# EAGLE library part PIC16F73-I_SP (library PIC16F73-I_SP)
8-bit CMOS FLASH Microcontrollers Source: Datasheet
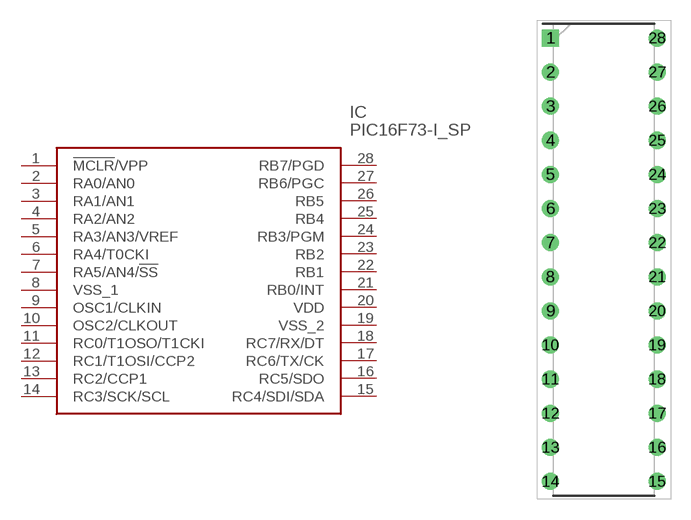
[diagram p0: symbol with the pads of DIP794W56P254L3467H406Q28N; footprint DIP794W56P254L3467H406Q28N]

Designator prefix IC

## PIC16F73-I_SP (Description: 8-bit CMOS FLASH Microcontrollers; Height: 4.06mm; Manufacturer_Name: Microchip; Manufacturer_Part_Number: PIC16F73-I/SP; Mouser_Part_Number: 579-PIC16F73ISP; Mouser_Price-Stock: https://www.mouser.co.uk/ProductDetail/Microchip-Technology-Atmel/PIC16F73-I-SP?qs=BJWliqx2vnXd6B3M0zIKjg%3D%3D)  [DIP794W56P254L3467H406Q28N]
1  !MCLR!/VPP
2  RA0/AN0
3  RA1/AN1
4  RA2/AN2
5  RA3/AN3/VREF
6  RA4/T0CKI
7  RA5/AN4/!SS
8  VSS_1
9  OSC1/CLKIN
10  OSC2/CLKOUT
11  RC0/T1OSO/T1CKI
12  RC1/T1OSI/CCP2
13  RC2/CCP1
14  RC3/SCK/SCL
15  RC4/SDI/SDA
16  RC5/SDO
17  RC6/TX/CK
18  RC7/RX/DT
19  VSS_2
20  VDD
21  RB0/INT
22  RB1
23  RB2
24  RB3/PGM
25  RB4
26  RB5
27  RB6/PGC
28  RB7/PGD

## Footprint DIP794W56P254L3467H406Q28N (pad centres in mm)
28 PDIP
drill 0.76 pad 1.16 square: 1 -3.97,16.51
drill 0.76 pad 1.16: 2 -3.97,13.97; 3 -3.97,11.43; 4 -3.97,8.89; 5 -3.97,6.35; 6 -3.97,3.81; 7 -3.97,1.27; 8 -3.97,-1.27; 9 -3.97,-3.81; 10 -3.97,-6.35; 11 -3.97,-8.89; 12 -3.97,-11.43; 13 -3.97,-13.97; 14 -3.97,-16.51; 15 3.97,-16.51; 16 3.97,-13.97; 17 3.97,-11.43; 18 3.97,-8.89; 19 3.97,-6.35; 20 3.97,-3.81; 21 3.97,-1.27; 22 3.97,1.27; 23 3.97,3.81; 24 3.97,6.35; 25 3.97,8.89; 26 3.97,11.43; 27 3.97,13.97; 28 3.97,16.51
